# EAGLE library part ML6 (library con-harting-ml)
HARTING
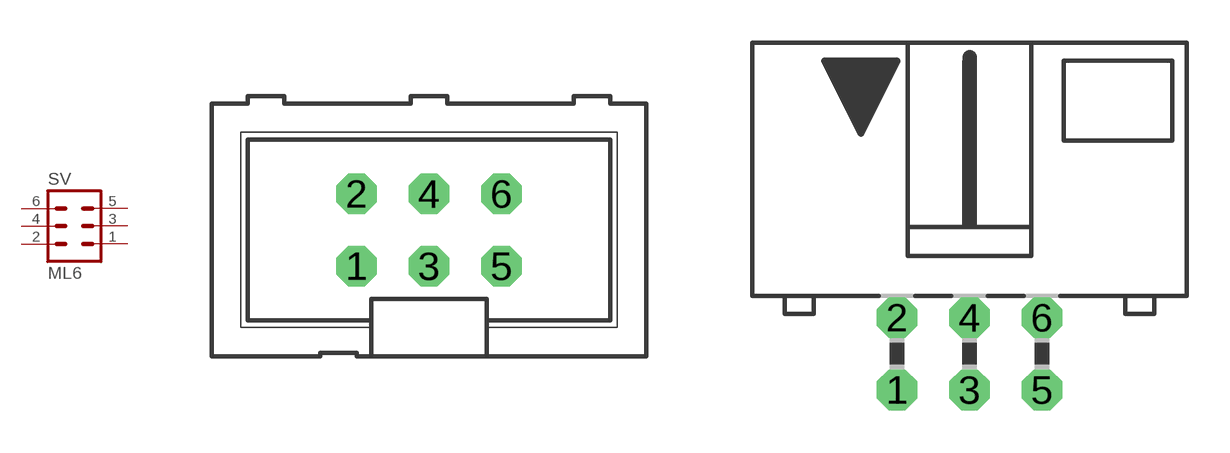
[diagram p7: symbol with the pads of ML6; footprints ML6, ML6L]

Designator prefix SV

## ML6 (OC_FARNELL: unknown; OC_NEWARK: unknown)  [ML6]
1  1  pas
2  2  pas
3  3  pas
4  4  pas
5  5  pas
6  6  pas

## ML6L (OC_FARNELL: unknown; OC_NEWARK: unknown)  [ML6L]
Pads as for ML6

## Footprint ML6 (pad centres in mm)
HARTING
drill 0.914 octagon: 1 -2.54,-1.27; 2 -2.54,1.27; 3 0,-1.27; 4 0,1.27; 5 2.54,-1.27; 6 2.54,1.27

## Footprint ML6L (pad centres in mm)
HARTING
drill 0.914 octagon: 1 -2.54,-1.27; 2 -2.54,1.27; 3 0,-1.27; 4 0,1.27; 5 2.54,-1.27; 6 2.54,1.27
